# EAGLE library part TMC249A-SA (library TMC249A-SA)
High Current Microstep Stepper Motor Driver with sensorless stall detection, protection / diagnosis and SPI Interface, SO-28
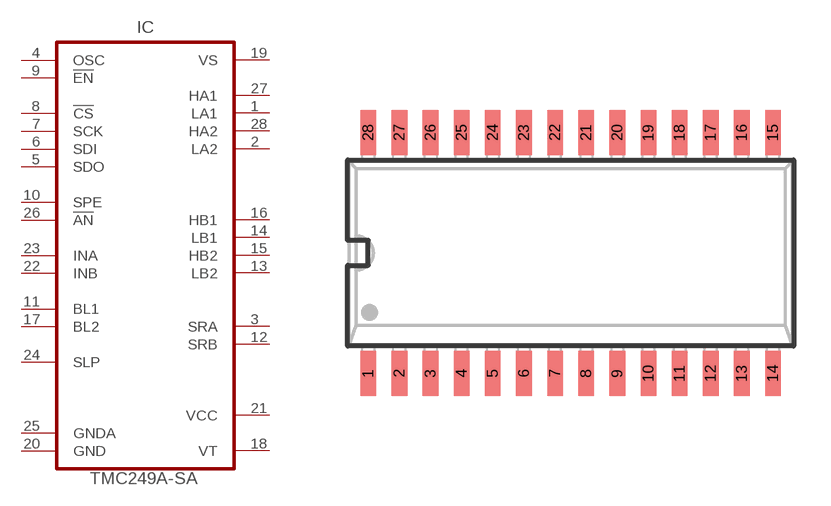
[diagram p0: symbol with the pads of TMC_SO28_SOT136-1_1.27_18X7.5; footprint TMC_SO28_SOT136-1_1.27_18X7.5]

Designator prefix IC

## TMC249A-SA (DATASHEET: http://www_trinamic_com/_scripts/download_php?file=_articles%2Fproducts%2Fintegrated-circuits%2Ftmc249%2F_datasheet%2FTMC249_datasheet_pdf; DESCRIPTION: High Current Microstep Stepper Motor Driver with sensorless stall detection, protection / diagnosis and SPI Interface, SO-28; DISTRIBUTOR1: Digikey; DISTRIBUTOR2: Farnell; GEOMETRY_HEIGHT: 2_65mm; MANUFACTURER: TRINAMIC; ORDERCODE-DISTRI1: 1460-10565-5-ND; ORDERCODE-DISTRI2: 1214193; ORDERCODE-MANU1: TMC249A-SA; VALUE: TMC249A-SA)  [TMC_SO28_SOT136-1_1.27_18X7.5]
1  LA1  out
2  LA2  out
3  SRA  in
4  OSC
5  SDO  out
6  SDI  in
7  SCK  in
8  !CS  in
9  !EN  in
10  SPE  in
11  BL1  in
12  SRB  in
13  LB2  out
14  LB1  out
15  HB2  out
16  HB1  out
17  BL2  in
18  VT  pwr
19  VS  pwr
20  GND  pwr
21  VCC  pwr
22  INB  in
23  INA  in
24  SLP  in
25  GNDA  pwr
26  !AN  in
27  HA1  out
28  HA2  out

## Footprint TMC_SO28_SOT136-1_1.27_18X7.5 (pad centres in mm)
smd 0.64 x 1.83: 1 -8.255,-4.912; 2 -6.985,-4.912; 3 -5.715,-4.912; 4 -4.445,-4.912; 5 -3.175,-4.912; 6 -1.905,-4.912; 7 -0.635,-4.912; 8 0.635,-4.912; 9 1.905,-4.912; 10 3.175,-4.912; 11 4.445,-4.912; 12 5.715,-4.912; 13 6.985,-4.912; 14 8.255,-4.912; 15 8.255,4.912; 16 6.985,4.912; 17 5.715,4.912; 18 4.445,4.912; 19 3.175,4.912; 20 1.905,4.912; 21 0.635,4.912; 22 -0.635,4.913; 23 -1.905,4.912; 24 -3.175,4.912; 25 -4.445,4.912; 26 -5.715,4.912; 27 -6.985,4.912; 28 -8.255,4.912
